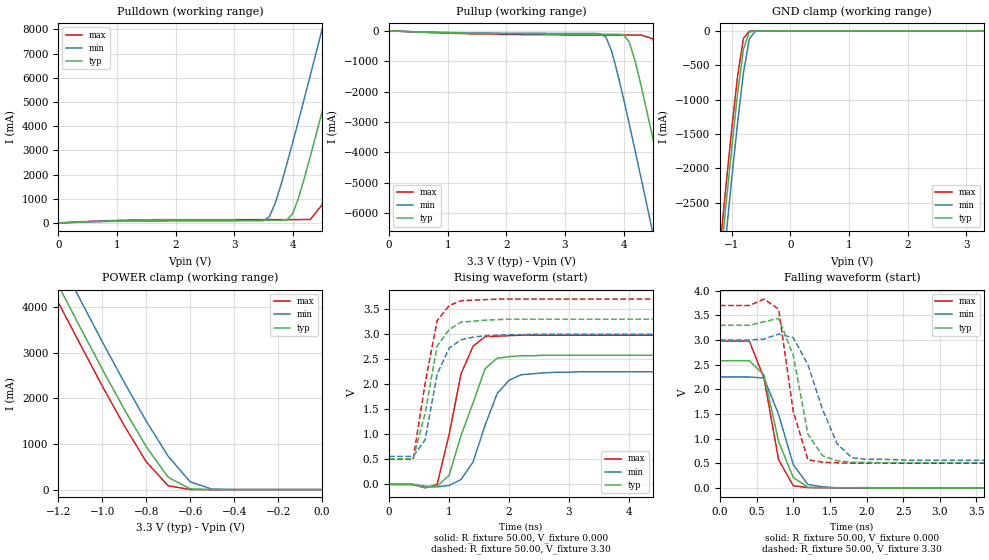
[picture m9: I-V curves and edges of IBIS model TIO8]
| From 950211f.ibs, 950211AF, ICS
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|   Model TIO8
[Model]   TIO8
Model_type   I/O
Polarity   Non-Inverting
Vinl =   0.80V
Vinh =   2.00V
C_comp   5.50pF   5.00pF   6.00pF
[Temperature Range]   27.00   70.00   0.000
[Voltage Range]   3.30V   3.00V   3.70V
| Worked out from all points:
|   slope of the pulldown table from 0 to 0.495 V, typ, clamps not added: 9.08 ohm
|   slope of the pullup table from 0 to 0.495 V, typ, clamps not added: 13.2 ohm
|   GND clamp passes 1 mA (typ) near -0.60 V on its own axis
|   POWER clamp passes 1 mA (typ) near -0.50 V on its own axis
|   rising waveform, R_fixture 50.00, V_fixture 0.000: 20-80 % time 444ps typ, 397ps min, 344ps max; typ from 0 V to 2.58 V
|   rising waveform, R_fixture 50.00, V_fixture 3.30: 20-80 % time 275ps typ, 296ps min, 282ps max; typ from 0.51 V to 3.3 V
|   falling waveform, R_fixture 50.00, V_fixture 0.000: 20-80 % time 283ps typ, 294ps min, 238ps max; typ from 2.58 V to 0 V
|   falling waveform, R_fixture 50.00, V_fixture 3.30: 20-80 % time 224ps typ, 359ps min, 229ps max; typ from 3.3 V to 0.51 V
[Pulldown]
| voltage   I(typ)   I(min)   I(max)
0V        7.1pA      1pA        22.2pA
3.5V      120mA      100mA      140mA
3.6V      120mA      260mA      140mA
3.7V      120mA      820mA      140mA
3.9V      130mA      2.45A      140mA
4V        390mA      3.34A      140mA
4.3V      2.76A      6.11A      150mA
4.5V      4.6A       8A         750mA
4.7V      6.48A      9.91A      2.42A
4.9V      8.38A      11.82A     4.25A
5.3V      12.22A     15.68A     8.04A
6.6V      24.9A      28.35A     20.68A
[Pullup]
| voltage   I(typ)   I(min)   I(max)
0V        260nA      170nA      390nA
3.7V      -110mA     -210mA     -140mA
3.8V      -110mA     -700mA     -140mA
4V        -130mA     -2.24A     -140mA
4.1V      -380mA     -3.1A      -140mA
4.3V      -1.82A     -4.87A     -140mA
4.5V      -3.55A     -6.67A     -260mA
4.7V      -5.34A     -8.5A      -1.57A
4.9V      -7.16A     -10.34A    -3.29A
5.1V      -9A        -12.19A    -5.09A
5.3V      -10.85A    -14.05A    -6.92A
6.6V      -23A       -26.21A    -19.02A
[GND_clamp]
| voltage   I(typ)   I(min)   I(max)
-3.3V     -22.88A    -23.3A     -22.62A
-1.2V     -3.43A     -3.89A     -3.15A
-1.1V     -2.55A     -3.01A     -2.27A
-1V       -1.71A     -2.15A     -1.43A
-900mV    -910mA     -1.34A     -660mA
-800mV    -270mA     -610mA     -110mA
-700mV    -17.7mA    -120mA     -4.49mA
-600mV    -940uA     -7.06mA    -460uA
-500mV    -76.73uA   -370uA     -37.56uA
3.3V      120pA      11.89uA    90.98pA
[POWER_clamp]
| voltage   I(typ)   I(min)   I(max)
-3.3V     24.71A     25.28A     24.35A
-1.3V     5.41A      6.02A      5.04A
-1.2V     4.48A      5.08A      4.1A
-1.1V     3.55A      4.16A      3.18A
-1V       2.64A      3.24A      2.27A
-900mV    1.76A      2.35A      1.4A
-800mV    940mA      1.5A       610mA
-700mV    270mA      730mA      83.95mA
-600mV    15.59mA    170mA      1.71mA
-500mV    350uA      9.94mA     24.64uA
0V        120pA      220pA      130pA
[Ramp]
| variable   typ   min   max
dV/dt_r   1.55/0.36n   1.35/0.40n   1.79/0.30n
dV/dt_f   1.67/0.19n   1.46/0.28n   1.92/0.17n
R_load = 50.00
[Rising Waveform]
R_fixture = 50.00
V_fixture = 0.000
V_fixture_min = 0.000
V_fixture_max = 0.000
| time   V(typ)   V(min)   V(max)
0s        0V         0V         0V
800ps     -36mV      -49.1mV    -3.21mV
1ns       180mV      -20.92mV   1V
1.2ns     980mV      98.43mV    2.21V
1.4ns     1.63V      450mV      2.76V
1.6ns     2.31V      1.18V      2.95V
1.8ns     2.52V      1.81V      2.96V
2ns       2.55V      2.08V      2.97V
2.2ns     2.57V      2.19V      2.98V
10ns      2.58V      2.25V      2.98V
[Rising Waveform]
R_fixture = 50.00
V_fixture = 3.30
V_fixture_min = 3.00
V_fixture_max = 3.70
| time   V(typ)   V(min)   V(max)
0s        510mV      560mV      500mV
400ps     510mV      560mV      500mV
600ps     1.42V      890mV      2.02V
800ps     2.76V      2.2V       3.27V
1ns       3.09V      2.72V      3.57V
1.2ns     3.24V      2.89V      3.67V
1.4ns     3.26V      2.94V      3.68V
1.6ns     3.28V      2.97V      3.69V
2.4ns     3.3V       3V         3.7V
10ns      3.3V       3V         3.7V
[Falling Waveform]
R_fixture = 50.00
V_fixture = 0.000
V_fixture_min = 0.000
V_fixture_max = 0.000
| time   V(typ)   V(min)   V(max)
0s        2.58V      2.25V      2.98V
400ps     2.58V      2.25V      2.98V
600ps     2.29V      2.23V      2.23V
800ps     940mV      1.49V      570mV
1ns       210mV      470mV      43.74mV
1.2ns     13.01mV    67.82mV    4.8mV
1.4ns     4.02mV     22.13mV    2.5mV
1.6ns     1.75mV     290uV      1.03mV
10ns      9.76uV     12.77uV    -1.03uV
[Falling Waveform]
R_fixture = 50.00
V_fixture = 3.30
V_fixture_min = 3.00
V_fixture_max = 3.70
| time   V(typ)   V(min)   V(max)
0s        3.3V       3V         3.7V
400ps     3.3V       3V         3.7V
600ps     3.37V      3.02V      3.83V
800ps     3.44V      3.12V      3.63V
1ns       2.69V      3.05V      1.55V
1.2ns     1.09V      2.5V       570mV
1.4ns     650mV      1.59V      520mV
1.6ns     550mV      890mV      510mV
1.8ns     520mV      610mV      500mV
10ns      510mV      560mV      500mV
